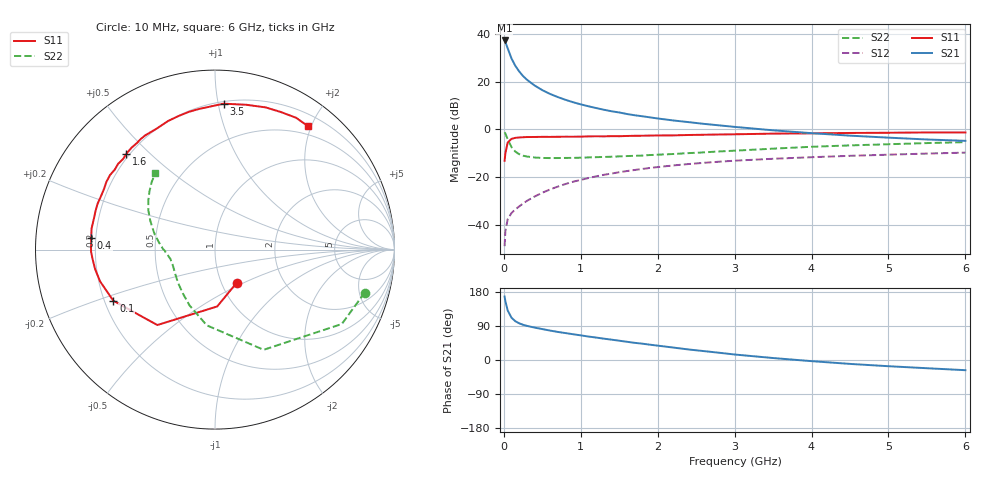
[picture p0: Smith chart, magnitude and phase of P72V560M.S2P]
! SIEMENS Small Signal Semiconductors
! BFP196
! Si NPN RF Bipolar Junction Transistor in SOT143
! VCE = 2.5 V  IC = 60 mA
! Common Emitter S-Parameters:  May  1996
# GHz  S  MA  R  50
!  f  S11  S21  S12  S22
! GHz  MAG  ANG  MAG  ANG  MAG  ANG  MAG  ANG
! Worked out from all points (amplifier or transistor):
!   36 points, 10 MHz to 6 GHz, reference 50 ohm
!   highest |S21| = 37.2 dB at 10 MHz (marker M1)
!   |S21| within 3 dB of that: start of sweep to 46.68 MHz
!   unconditionally stable (mu >= 1): 391.4 MHz to 4.43 GHz
!   at 250 MHz: K = 0.89, MSG = 26.7 dB, |S12| = -31.0 dB
!   at 1.4 GHz: K = 1.09, MAG = 11.2 dB, |S12| = -18.5 dB
!   at 6 GHz: K = 0.98, MSG = 2.5 dB, |S12| = -9.7 dB
!   S11 on the Smith chart (normalised r, x): 10 MHz: 1.18, -0.46; 100 MHz: 0.24, -0.22; 400 MHz: 0.18, +0.04; 1.6 GHz: 0.19, +0.43; 3.5 GHz: 0.21, +1.04; 6 GHz: 0.37, +1.95
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0.01  0.2211 -57.0  72.46 167.4  0.0036 77.8  0.8682 -16.0
0.02  0.317 -87.8  67.39 155.0  0.0074 71.1  0.8192 -30.4
0.05  0.5291 -127.4  49.59 130.7  0.0132 55.1  0.6206 -64.1
0.1  0.6341 -153.3  30.34 111.5  0.0178 50.4  0.4244 -96.2
0.15  0.6645 -164.6  21.26 102.2  0.0212 51.0  0.3419 -114.5
0.2  0.6769 -170.8  16.25 96.8  0.0245 55.0  0.3025 -126.4
0.25  0.6848 -176.0  13.03 92.9  0.0281 57.0  0.2812 -135.5
0.3  0.6908 -179.2  10.93 90.1  0.0319 59.2  0.2702 -141.5
0.4  0.6929 174.7  8.276 85.5  0.0394 62.2  0.2576 -150.4
0.5  0.6977 170.3  6.62 81.6  0.0472 63.5  0.2524 -156.1
0.6  0.6963 166.1  5.519 77.7  0.0553 63.9  0.2508 -159.9
0.7  0.6996 162.1  4.747 74.1  0.0634 64.3  0.2512 -162.9
0.9  0.7015 154.8  3.697 68.0  0.0803 62.7  0.253 -167.4
1.1  0.7131 148.1  3.04 61.9  0.0959 61.1  0.2588 -170.5
1.3  0.7143 141.5  2.575 56.3  0.1121 58.3  0.2647 -173.4
1.6  0.7276 132.7  2.096 48.1  0.1344 54.5  0.2763 -177.0
2.2  0.7482 115.8  1.538 32.9  0.1757 45.4  0.305 175.1
2.8  0.7812 100.7  1.213 19.1  0.2107 36.5  0.3454 166.0
3.5  0.8145 86.6  0.955 5.2  0.2426 26.5  0.3951 155.9
4.5  0.8411 70.4  0.739 -10.3  0.2797 14.5  0.4622 143.4
5.5  0.8623 58.4  0.614 -21.7  0.3116 3.6  0.5165 133.0
6  0.861 53.0  0.576 -26.9  0.3262 -2.1  0.5413 127.9
